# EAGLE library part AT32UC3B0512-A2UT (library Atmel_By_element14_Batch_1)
32-bit AVR® Microcontroller
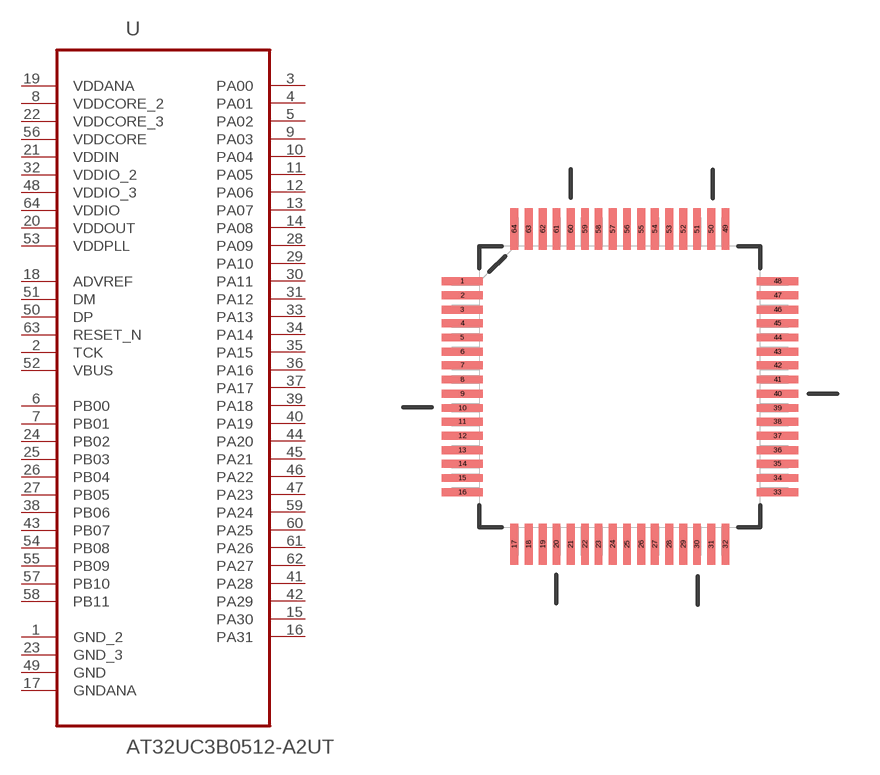
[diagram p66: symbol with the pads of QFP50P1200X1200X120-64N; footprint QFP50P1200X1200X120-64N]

Designator prefix U

## AT32UC3B0512-A2UT (DESCRIPTION: 32-bit AVR® Microcontroller; MPN: AT32UC3B0512-A2UT; OC_FARNELL: 1841640; OC_NEWARK: 12T1373; PACKAGE: QFP-64; SUPPLIER: Atmel)  [QFP50P1200X1200X120-64N]
1  GND_2  pas
2  TCK  in
3  PA00
4  PA01
5  PA02
6  PB00
7  PB01
8  VDDCORE_2  pwr
9  PA03
10  PA04
11  PA05
12  PA06
13  PA07
14  PA08
15  PA30
16  PA31
17  GNDANA  pas
18  ADVREF  in
19  VDDANA  pwr
20  VDDOUT  pwr
21  VDDIN  pwr
22  VDDCORE_3  pwr
23  GND_3  pas
24  PB02
25  PB03
26  PB04
27  PB05
28  PA09
29  PA10
30  PA11
31  PA12
32  VDDIO_2  pwr
33  PA13
34  PA14
35  PA15
36  PA16
37  PA17
38  PB06
39  PA18
40  PA19
41  PA28
42  PA29
43  PB07
44  PA20
45  PA21
46  PA22
47  PA23
48  VDDIO_3  pwr
49  GND  pas
50  DP  pas
51  DM  pas
52  VBUS  in
53  VDDPLL  pwr
54  PB08
55  PB09
56  VDDCORE  pwr
57  PB10
58  PB11
59  PA24
60  PA25
61  PA26
62  PA27
63  RESET_N  in
64  VDDIO  pwr

## Footprint QFP50P1200X1200X120-64N (pad centres in mm)
smd 1.473 x 0.279: 1 -5.613,3.759; 2 -5.613,3.251; 3 -5.613,2.743; 4 -5.613,2.261; 5 -5.613,1.753; 6 -5.613,1.245; 7 -5.613,0.762; 8 -5.613,0.254; 9 -5.613,-0.254; 10 -5.613,-0.762; 11 -5.613,-1.245; 12 -5.613,-1.753; 13 -5.613,-2.261; 14 -5.613,-2.743; 15 -5.613,-3.251; 16 -5.613,-3.759; 33 5.613,-3.759; 34 5.613,-3.251; 35 5.613,-2.743; 36 5.613,-2.261; 37 5.613,-1.753; 38 5.613,-1.245; 39 5.613,-0.762; 40 5.613,-0.254; 41 5.613,0.254; 42 5.613,0.762; 43 5.613,1.245; 44 5.613,1.753; 45 5.613,2.261; 46 5.613,2.743; 47 5.613,3.251; 48 5.613,3.759
smd 0.279 x 1.473: 17 -3.759,-5.613; 18 -3.251,-5.613; 19 -2.743,-5.613; 20 -2.261,-5.613; 21 -1.753,-5.613; 22 -1.245,-5.613; 23 -0.762,-5.613; 24 -0.254,-5.613; 25 0.254,-5.613; 26 0.762,-5.613; 27 1.245,-5.613; 28 1.753,-5.613; 29 2.261,-5.613; 30 2.743,-5.613; 31 3.251,-5.613; 32 3.759,-5.613; 49 3.759,5.613; 50 3.251,5.613; 51 2.743,5.613; 52 2.261,5.613; 53 1.753,5.613; 54 1.245,5.613; 55 0.762,5.613; 56 0.254,5.613; 57 -0.254,5.613; 58 -0.762,5.613; 59 -1.245,5.613; 60 -1.753,5.613; 61 -2.261,5.613; 62 -2.743,5.613; 63 -3.251,5.613; 64 -3.759,5.613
